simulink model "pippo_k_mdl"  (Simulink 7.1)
settings: Solver=ode45  StartTime=0.0  StopTime=10.0  RelTol=1e-3
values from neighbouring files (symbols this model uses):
  bm = 0.02*N*m*sec/rad    (= 0.02)    [pippo.m]
  Cr = 0*N*m    (= 0)    [pippo.m]
  Ia_0 = 0*A    (= 0)    [pippo.m]
  Ia_max = 10000000*A    (= 10000000)    [pippo.m]
  Jm = 0.5*Kg*m^2    (= 0.5)    [pippo.m]
  K = (1/Ep-1)/dcgain(gs)    [pippo.m]
  Km = 1    [pippo.m]
  La = 10*mHenry    (= 0.01)    [pippo.m]
  Ra = 2*Ohm    (= 2)    [pippo.m]
  tau1 = 0    [pippo.m]
  tau2 = 0    [pippo.m]
  Tc = Tfin/2000    (= 5e-05)    [pippo.m]
  Va_max = 10000000*V    (= 10000000)    [pippo.m]
  Wm_0 = 0*rpm    (= 0)    [pippo.m]
  Wref = 600*rpm    (= 62.8318530718)    [pippo.m]

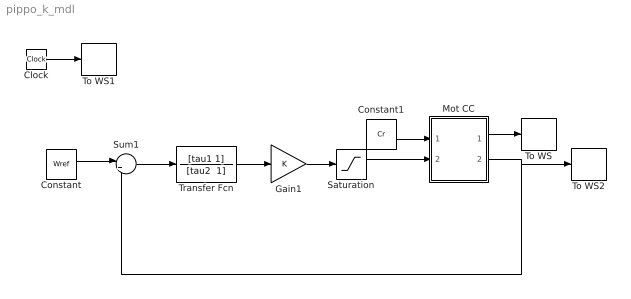
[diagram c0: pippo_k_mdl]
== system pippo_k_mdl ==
  Clock : Clock
  Constant : Constant  Value=Wref  OutDataType=sfix(16)  OutScaling=2^0
  Constant1 : Constant  Value=Cr  OutDataType=sfix(16)  OutScaling=2^0
  Gain1 : Gain  Gain=K  ParameterDataType=sfix(16)  ParameterScaling=2^0  OutDataType=sfix(16)  OutScaling=2^0
  Mot CC : Subsystem
  Saturation : Saturate  UpperLimit=Va_max  LowerLimit=-Va_max  OutDataType=sfix(16)  OutScaling=2^0
  Sum1 : Sum  Inputs=|+-  OutDataType=sfix(16)  OutScaling=2^0
  To WS : ToWorkspace  VariableName=Ia  SampleTime=Tc  SaveFormat=Array
  To WS1 : ToWorkspace  VariableName=t  SampleTime=Tc  SaveFormat=Array
  To WS2 : ToWorkspace  VariableName=Wm  SampleTime=Tc  SaveFormat=Array
  Transfer Fcn : TransferFcn  Numerator=[tau1 1]  Denominator="[tau2  1]"
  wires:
  Clock/1 -> To WS1/1
  Constant1/1 -> Mot CC/1(Tr)
  Mot CC/1(Ia) -> To WS/1
  Mot CC/2(Wm) -> To WS2/1, Sum1/2
  Constant/1 -> Sum1/1
  Sum1/1 -> Transfer Fcn/1
  Gain1/1 -> Saturation/1
  Saturation/1 -> Mot CC/2(Va)
  Transfer Fcn/1 -> Gain1/1

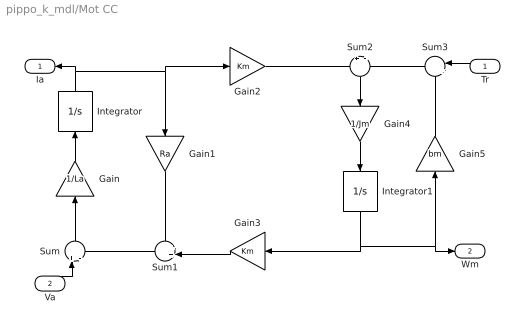
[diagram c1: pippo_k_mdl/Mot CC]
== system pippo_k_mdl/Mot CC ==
  Tr : Inport  Orientation=left
  Va : Inport  Orientation=up  Port=2
  Gain : Gain  Orientation=up  Gain=1/La  ParameterDataType=sfix(16)  ParameterScaling=2^0  OutDataType=sfix(16)  OutScaling=2^0
  Gain1 : Gain  Orientation=down  Gain=Ra  ParameterDataType=sfix(16)  ParameterScaling=2^0  OutDataType=sfix(16)  OutScaling=2^0
  Gain2 : Gain  Gain=Km  ParameterDataType=sfix(16)  ParameterScaling=2^0  OutDataType=sfix(16)  OutScaling=2^0
  Gain3 : Gain  Orientation=left  Gain=Km  ParameterDataType=sfix(16)  ParameterScaling=2^0  OutDataType=sfix(16)  OutScaling=2^0
  Gain4 : Gain  Orientation=down  Gain=1/Jm  ParameterDataType=sfix(16)  ParameterScaling=2^0  OutDataType=sfix(16)  OutScaling=2^0
  Gain5 : Gain  Orientation=up  Gain=bm  ParameterDataType=sfix(16)  ParameterScaling=2^0  OutDataType=sfix(16)  OutScaling=2^0
  Integrator : Integrator  Orientation=up  InitialCondition=Ia_0  LimitOutput=on  UpperSaturationLimit=Ia_max  LowerSaturationLimit=-Ia_max
  Integrator1 : Integrator  Orientation=down  InitialCondition=Wm_0
  Sum : Sum  Orientation=up  Inputs=+|-  OutDataType=sfix(16)  OutScaling=2^0
  Sum1 : Sum  Orientation=left  Inputs=++|  OutDataType=sfix(16)  OutScaling=2^0
  Sum2 : Sum  Orientation=down  Inputs=+|-  OutDataType=sfix(16)  OutScaling=2^0
  Sum3 : Sum  Orientation=left  Inputs=|++  OutDataType=sfix(16)  OutScaling=2^0
  Ia : Outport  Orientation=left
  Wm : Outport  Port=2
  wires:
  Sum/1 -> Gain/1
  Gain/1 -> Integrator/1
  Integrator/1 -> Gain1/1, Gain2/1, Ia/1
  Sum1/1 -> Sum/2
  Gain1/1 -> Sum1/1
  Gain3/1 -> Sum1/2
  Gain2/1 -> Sum2/1
  Sum2/1 -> Gain4/1
  Gain4/1 -> Integrator1/1
  Integrator1/1 -> Gain3/1, Gain5/1, Wm/1
  Gain5/1 -> Sum3/2
  Sum3/1 -> Sum2/2
  Tr/1 -> Sum3/1
  Va/1 -> Sum/1
